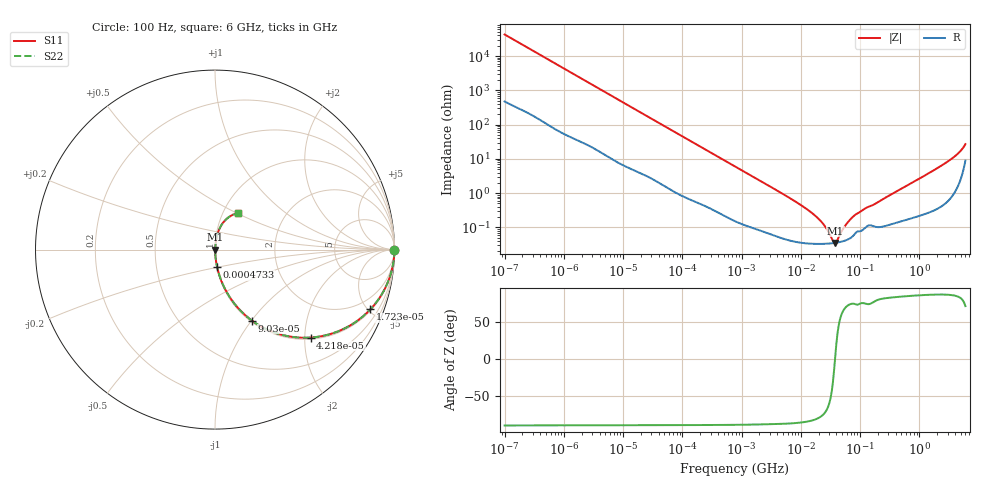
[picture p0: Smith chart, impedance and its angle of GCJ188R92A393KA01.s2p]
!Murata Part Number: GCJ188R92A393KA01
!These Parameters are Measured in Series Mode Connection
!Data Generated on Mar 13, 2026
!  o--ll--o
!Port1  Port2
!  o------o
!Operation Temp=25[degC], DC Bias Voltage=0[V]
!Freq. Start=100[Hz] Stop=6[GHz] 401[Steps]
# Hz S RI R 50
!Freq.(Hz) S11(Real) S11(Imag) S21(Real) S21(Imag) S12(Real) S12(Imag) S22(Real) S22(Imag)
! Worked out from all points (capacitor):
!   401 points, 100 Hz to 6 GHz, reference 50 ohm
!   read as one part in series: C = 37.1 nF near 109 Hz
!   lowest |Z| = 35.5 mohm at 38.09 MHz (marker M1)
!   series resonance near 37.82 MHz, so ESL is about 480 pH
!   S11 on the Smith chart (normalised r, x): 100 Hz: open; 17.23 kHz: 1.09, -5.18; 42.18 kHz: 1.04, -2.14; 90.3 kHz: 1.02, -1.01; 473.3 kHz: 1.00, -0.20; 6 GHz: 1.18, +0.51
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100  1 -0.00234  3.15e-05 0.00234  3.15e-05 0.00234  1 -0.00234
2008  0.9973 -0.0458  0.00275 0.0458  0.00275 0.0458  0.9973 -0.0458
6433  0.9773 -0.1418  0.0227 0.1418  0.0227 0.1418  0.9773 -0.1418
17227  0.8662 -0.3323  0.1338 0.3323  0.1338 0.3323  0.8662 -0.3323
40335  0.5546 -0.4881  0.4454 0.4881  0.4454 0.4881  0.5546 -0.4881
42182  0.533 -0.49  0.467 0.49  0.467 0.49  0.533 -0.49
90302  0.2064 -0.3959  0.7936 0.3959  0.7936 0.3959  0.2064 -0.3959
176758  0.0672 -0.2403  0.9328 0.2403  0.9328 0.2403  0.0672 -0.2403
473344  0.0118 -0.0967  0.9882 0.0967  0.9882 0.0967  0.0118 -0.0967
774597  0.00512 -0.0599  0.9949 0.0599  0.9949 0.0599  0.00512 -0.0599
6353432  0.000473 -0.00737  0.9995 0.00737  0.9995 0.00737  0.000473 -0.00737
1.555665e7  0.00034 -0.00259  0.9997 0.00259  0.9997 0.00259  0.00034 -0.00259
2.327686e7  0.000333 -0.00129  0.9997 0.00129  0.9997 0.00129  0.000333 -0.00129
3.482834e7  0.000348 -0.000212  0.9997 0.000212  0.9997 0.000212  0.000348 -0.000212
3.80911e7  0.000355 1.88e-05  0.9996 -1.88e-05  0.9996 -1.88e-05  0.000355 1.88e-05
4.165952e7  0.000364 0.00025  0.9996 -0.00025  0.9996 -0.00025  0.000364 0.00025
5.699437e7  0.00042 0.00109  0.9996 -0.00109  0.9996 -0.00109  0.00042 0.00109
7.797396e7  0.000593 0.00206  0.9994 -0.00206  0.9994 -0.00206  0.000593 0.00206
3.124326e8  0.00126 0.0085  0.9987 -0.0085  0.9987 -0.0085  0.00126 0.0085
2.679998e9  0.01 0.072  0.99 -0.072  0.99 -0.072  0.01 0.072
4.586474e9  0.0371 0.1388  0.9629 -0.1388  0.9629 -0.1388  0.0371 0.1388
6e9  0.1293 0.2041  0.8707 -0.2041  0.8707 -0.2041  0.1293 0.2041
